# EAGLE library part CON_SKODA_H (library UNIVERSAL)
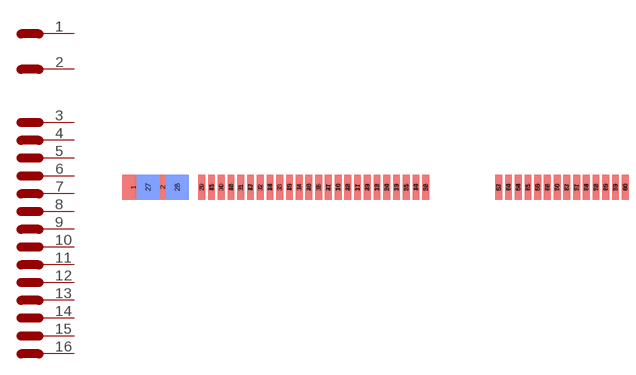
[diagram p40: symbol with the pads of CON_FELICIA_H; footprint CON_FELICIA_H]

Designator prefix CON; gates G$1=PIN G$2=PIN G$3=PIN G$4=PIN G$5=PIN G$6=PIN G$7=PIN G$8=PIN G$9=PIN G$10=PIN G$11=PIN G$12=PIN G$13=PIN G$14=PIN G$15=PIN G$16=PIN G$17=PIN G$18=PIN G$19=PIN G$20=PIN G$21=PIN G$22=PIN G$23=PIN G$24=PIN G$25=PIN G$26=PIN G$27=PIN G$28=PIN G$29=PIN G$30=PIN G$31=PIN G$32=PIN G$33=PIN G$34=PIN G$35=PIN G$36=PIN G$37=PIN G$38=PIN G$39=PIN G$40=PIN G$41=PIN G$42=PIN G$43=PIN G$44=PIN G$45=PIN G$46=PIN G$47=PIN G$48=PIN G$49=PIN G$50=PIN G$51=PIN G$52=PIN G$53=PIN G$54=PIN G$55=PIN G$56=PIN G$57=PIN G$58=PIN G$59=PIN G$60=PIN G$61=PIN G$62=PIN G$63=PIN G$64=PIN G$65=PIN G$66=PIN G$67=PIN G$68=PIN G$69=PIN G$70=PIN G$71=PIN G$72=PIN G$73=PIN G$74=PIN G$75=PIN G$76=PIN G$77=PIN G$78=PIN G$79=PIN G$80=PIN

## CON_SKODA_H  [CON_FELICIA_H]
1  G$1:1
2  G$2:1
3  G$3:1
4  G$4:1
5  G$5:1
6  G$6:1
7  G$7:1
8  G$8:1
9  G$9:1
10  G$10:1
11  G$11:1
12  G$12:1
13  G$13:1
14  G$14:1
15  G$15:1
16  G$16:1
17  G$17:1
18  G$18:1
19  G$19:1
20  G$20:1
21  G$21:1
22  G$22:1
23  G$23:1
24  G$24:1
25  G$25:1
26  G$26:1
27  G$27:1
28  G$28:1
29  G$29:1
30  G$30:1
31  G$31:1
32  G$32:1
33  G$33:1
34  G$34:1
35  G$35:1
36  G$36:1
37  G$37:1
38  G$38:1
39  G$39:1
40  G$40:1
41  G$41:1
42  G$42:1
43  G$43:1
44  G$44:1
45  G$45:1
46  G$46:1
47  G$47:1
48  G$48:1
49  G$49:1
50  G$50:1
51  G$51:1
52  G$52:1
53  G$53:1
54  G$54:1
55  G$55:1
56  G$56:1
57  G$57:1
58  G$58:1
59  G$59:1
60  G$60:1
61  G$61:1
62  G$62:1
63  G$63:1
64  G$64:1
65  G$65:1
66  G$66:1
67  G$67:1
68  G$68:1
69  G$69:1
70  G$70:1
71  G$71:1
72  G$72:1
73  G$73:1
74  G$74:1
75  G$75:1
76  G$76:1
77  G$77:1
78  G$78:1
79  G$79:1
80  G$80:1

## Footprint CON_FELICIA_H (pad centres in mm)
smd 5 x 5.5: 1 -14.98,0.535; 2 -8.56,0.535
smd 1.5 x 5.5 bottom: 3 0,0.535; 4 4.28,0.535; 5 8.56,0.535; 6 12.84,0.535; 7 17.12,0.535; 8 21.4,0.535; 9 25.68,0.535; 10 29.96,0.535; 11 34.24,0.535; 12 38.52,0.535; 13 42.8,0.535; 14 47.08,0.535; 15 2.14,0.535; 16 6.42,0.535; 17 10.7,0.535; 18 14.98,0.535; 19 19.26,0.535; 20 23.54,0.535; 21 27.82,0.535; 22 32.1,0.535; 23 36.38,0.535; 24 40.66,0.535; 25 44.94,0.535; 26 49.22,0.535; 53 65.27,0.535; 54 69.55,0.535; 55 73.83,0.535; 56 78.11,0.535; 57 82.39,0.535; 58 86.67,0.535; 59 90.95,0.535; 60 67.41,0.535; 61 71.69,0.535; 62 75.97,0.535; 63 80.25,0.535; 64 84.53,0.535; 65 88.81,0.535; 66 93.09,0.535
smd 5 x 5.5 bottom: 27 -11.77,0.535; 28 -5.35,0.535
smd 1.5 x 5.5: 29 0,0.535; 30 4.28,0.535; 31 8.56,0.535; 32 12.84,0.535; 33 17.12,0.535; 34 21.4,0.535; 35 25.68,0.535; 36 29.96,0.535; 37 34.24,0.535; 38 38.52,0.535; 39 42.8,0.535; 40 47.08,0.535; 41 2.14,0.535; 42 6.42,0.535; 43 10.7,0.535; 44 14.98,0.535; 45 19.26,0.535; 46 23.54,0.535; 47 27.82,0.535; 48 32.1,0.535; 49 36.38,0.535; 50 40.66,0.535; 51 44.94,0.535; 52 49.22,0.535; 67 65.27,0.535; 68 69.55,0.535; 69 73.83,0.535; 70 78.11,0.535; 71 82.39,0.535; 72 86.67,0.535; 73 90.95,0.535; 74 67.41,0.535; 75 71.69,0.535; 76 75.97,0.535; 77 80.25,0.535; 78 84.53,0.535; 79 88.81,0.535; 80 93.09,0.535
